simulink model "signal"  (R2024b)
settings: Solver=VariableStepAuto  StartTime=0.0  StopTime=8  RelTol=1e-3
libraries: simulink x2

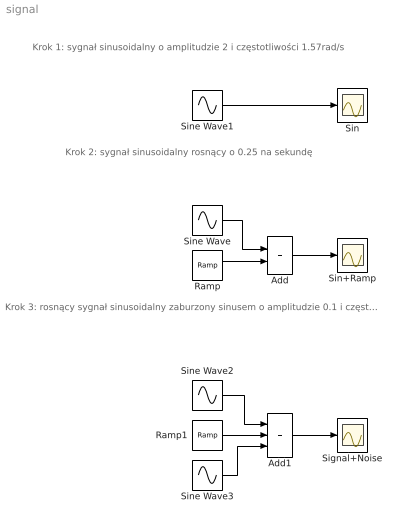
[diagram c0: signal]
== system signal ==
  note: Krok 1: sygnał sinusoidalny o amplitudzie 2 i częstotliwości 1.57rad/s
  note: Krok 2: sygnał sinusoidalny rosnący o 0.25 na sekundę
  note: Krok 3: rosnący sygnał sinusoidalny zaburzony sinusem o amplitudzie 0.1 i częstotliwości 31 rad/s (ok. 20-krotnie wyższą niż częstotliwość właściwego sygnału)
  Add : Sum
  Add1 : Sum  Inputs=+++
  Ramp : simulink/Sources/Ramp  slope=0.25  start=0  InitialOutput=0
  Ramp1 : simulink/Sources/Ramp  slope=0.25  start=0  InitialOutput=0
  Signal+Noise : Scope
  Sin : Scope
  Sin+Ramp : Scope
  Sine Wave : Sin  Amplitude=2  Frequency=1.57  SampleTime=0
  Sine Wave1 : Sin  Amplitude=2  Frequency=1.57  SampleTime=0
  Sine Wave2 : Sin  Amplitude=2  Frequency=1.57  SampleTime=0
  Sine Wave3 : Sin  Amplitude=0.1  Frequency=31  SampleTime=0
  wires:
  Ramp/1 -> Add/2
  Sine Wave/1 -> Add/1
  Add/1 -> Sin+Ramp/1
  Sine Wave1/1 -> Sin/1
  Add1/1 -> Signal+Noise/1
  Ramp1/1 -> Add1/2
  Sine Wave2/1 -> Add1/1
  Sine Wave3/1 -> Add1/3
